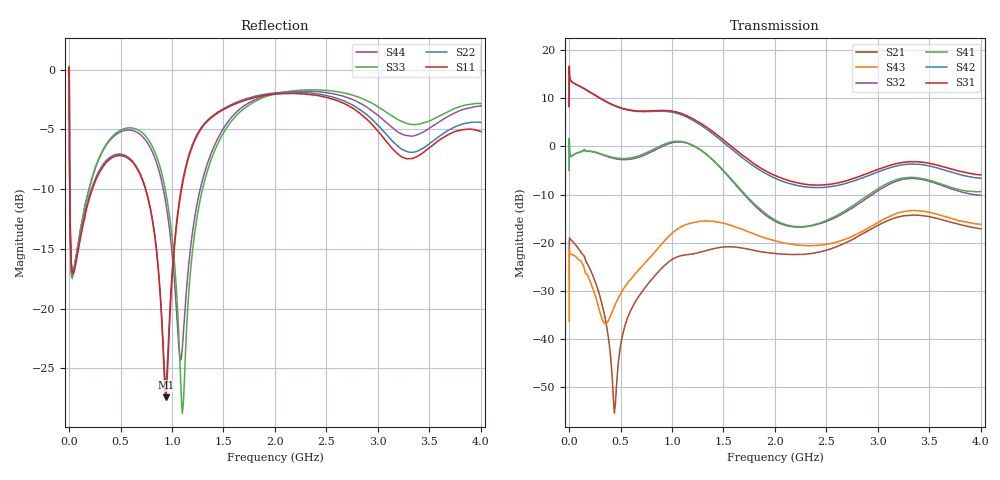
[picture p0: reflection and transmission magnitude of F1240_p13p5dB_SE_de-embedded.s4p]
! Integrated Device Technology
! Corporate Headquarters
! 6024 Silver Creek Valley Road
! San Jose, CA 95138  USA
! Phone:  1-408-284-8200
! Toll Free:  1-800-223-1366
! Webpage:  http://www.idt.com/
! Timing and RF Division
! 515 Groton Road, Suite 102
! Westford, MA 01886-6024
! Device:  F1240
! Description: Dual Intermediate Frequency Digital Variable Gain Amplifier
! Frequency:  10.0 -  500.00 MHz
! Package:  5x5 mm QFN Plastic Package: 32 pin
! Ports:  8 RF, 20 DC
!  Pin  1  = GA3 / Data  Pin 17  = RF OUT_B+
!  Pin  2  = GA4 / CLK  Pin 18  = RF OUT_B-
!  Pin  3  = GA5  Pin 19  = STBY_B
!  Pin  4  = VMODE  Pin 20  = Ground
!  Pin  5  = No Connect  Pin 21  = Ground
!  Pin  6  = GB5  Pin 22  = STB_A
!  Pin  7  = GB4  Pin 23  = RF OUT_A-  = Port 4
!  Pin  8  = GB3  Pin 24  = RF OUT_A+  = Port 3
!  Pin  9  = GB2  Pin 25  = GA0
!  Pin 10  = GB1  Pin 26  = ISET_A
!  Pin 11  = RF IN_B+  Pin 27  = VCC
!  Pin 12  = RF IN_B-  Pin 28  = Ground
!  Pin 13  = Ground  Pin 29  = RF IN_A-  = Port 2
!  Pin 14  = VCC  Pin 30  = RF IN_A+  = Port 1
!  Pin 15  = ISET_B  Pin 31  = GA1
!  Pin 16  = GB0  Pin 32  = GA2 / CSb
! Gain  = +19.5 dB
! State  = 1
! Voltage  = +5.00 V
! Current  = 85.292 mA (one channel only)
! Temperture  =  +25 C
! Test Date  =  2017-10-18
! Board  =  EB4031
! Data:  The device was measured on a custom evaluation board which has
!  individual transmission lines to the RF pins.  Data was collected
!  using a calibrated network analyzer.  The evaluation board was
!  de-embedded using Automatic Fixture Removal.
!  The reference plane is the edge of the package pin.
!  Only Channel A was measured.
!  This data is in single-ended operation.  If your needs are balanced
!  or differential S-parameters then this file needs to be used a
!  linear simulator.
! File Date:  2017-11-10  MJV
! Note:
!  Integrated Device Technology supplies this data as a sample of measured
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# Hz S dB R 100
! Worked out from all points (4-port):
!   410 points, 500 kHz to 4 GHz, reference 100 ohm
!   strongest paths, dB at 500 kHz, 930 MHz, 1.96 GHz, 2.98 GHz, 4 GHz:
!     S31: 8.3, 7.5, -5.6, -4.9, -5.9
!     S42: 8.3, 7.3, -6.2, -5.5, -6.6
!     S41: -4.9, 0.5, -14.7, -9.1, -9.4
!     S32: -4.9, 0.2, -15.0, -9.5, -10.1
!     S43: -36.3, -19.5, -19.3, -16.0, -16.2
!     S21: -27.6, -24.6, -22.1, -16.6, -17.1
!   lowest |S11| = -27.4 dB at 940 MHz (marker M1), VSWR 1.09, Z = 108 + j4.48 ohm
!   |S11| at or under -10 dB: 7.119 MHz to 226.5 MHz (219.4 MHz wide, 188 % of centre); 742.3 MHz to 1.093 GHz (350.3 MHz wide, 38.2 % of centre)
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500000  -0.35 -6.0  -27.54 1.7  -27.27 78.5  -60.14 66.5
        -27.59 1.2  -0.34 -5.9  -59.67 66.3  -27.28 79.6
        8.31 -105.2  -4.89 71.6  -0.44 1.2  -36.29 -143.7
        -4.91 72.8  8.29 -104.1  -36.28 -143.5  -0.45 3.5
3000000  -3.99 -58.3  -19.28 15.0  -17.93 17.2  -40.53 62.9
         -19.28 15.0  -3.95 -58.3  -40.48 62.9  -17.94 17.3
         15.95 -175.4  0.05 -9.1  -3.55 -54.0  -21.42 41.7
         0.06 -9.0  15.94 -175.1  -21.38 41.5  -3.61 -53.8
2e8  -10.70 -122.5  -25.19 -92.8  -20.48 -51.1  -34.31 8.4
     -25.26 -91.6  -10.48 -123.9  -34.28 8.8  -20.50 -51.1
     11.34 109.8  -1.02 -48.6  -9.81 -85.4  -27.16 -104.2
     -0.95 -48.8  11.30 109.0  -27.72 -101.5  -9.81 -84.5
5.4e8  -7.27 -176.3  -38.41 15.5  -22.04 -108.7  -28.20 -58.8
       -37.39 3.4  -7.16 -177.6  -28.33 -57.3  -22.18 -109.0
       7.79 24.6  -2.74 -122.7  -4.93 -153.5  -30.88 40.9
       -2.51 -124.0  7.70 23.6  -29.17 25.3  -5.09 -153.2
9.4e8  -27.41 29.2  -23.61 -66.8  -19.64 168.5  -23.97 -153.3
       -24.46 -77.5  -26.39 24.4  -24.27 -148.1  -20.02 167.9
       7.46 -74.1  0.33 147.4  -10.28 142.3  -20.37 -50.6
       0.59 142.9  7.28 -75.8  -19.27 -64.7  -11.19 145.6
1.52e9  -3.24 -148.2  -20.45 151.5  -25.40 32.7  -26.06 72.1
        -20.83 155.7  -3.17 -148.2  -25.89 77.8  -26.48 32.0
        1.01 124.2  -5.59 -35.5  -5.01 -133.3  -16.34 141.8
        -5.44 -40.6  0.49 122.9  -16.03 136.3  -4.64 -136.5
4e9  -5.18 -155.2  -17.12 65.6  -21.27 -50.4  -20.07 -48.3
     -17.07 65.0  -4.41 -150.1  -22.16 -29.1  -24.31 -39.8
     -5.89 9.9  -10.11 -115.4  -2.84 -137.5  -15.72 89.3
     -9.37 -127.0  -6.60 18.9  -16.16 62.5  -3.04 -143.3
